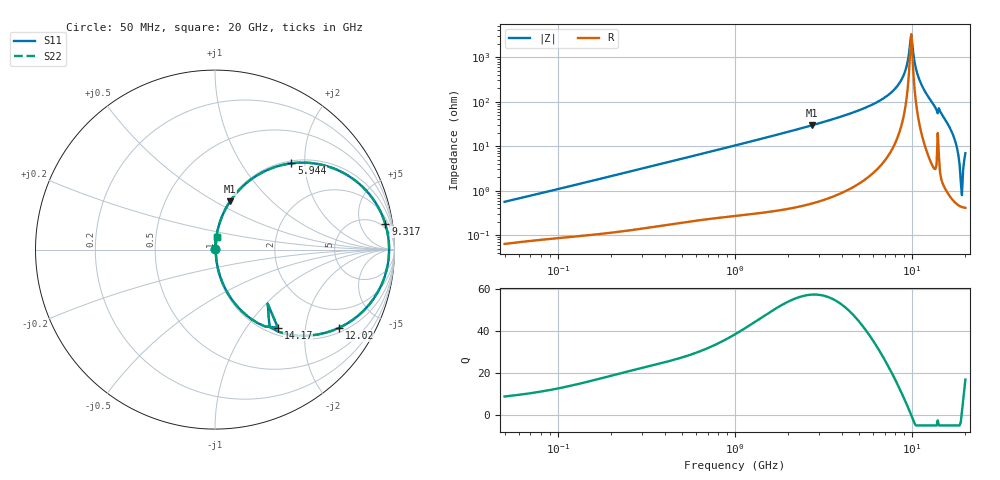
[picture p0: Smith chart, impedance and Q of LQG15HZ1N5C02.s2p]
!Murata Part Number: LQG15HZ1N5C02
!These Parameters are Measured in Series Mode Connection
!  o--[Z]--o
!Port1  Port2
!  o-------o
!Freq. Start=50[MHz] Stop=20[GHz], 401[Steps]
# Hz S RI R 50
!Freq.(Hz) S11(Real) S11(Imag) S21(Real) S21(Imag) S12(Real) S12(Imag) S22(Real) S22(Imag)
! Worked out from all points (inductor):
!   401 points, 50 MHz to 20 GHz, reference 50 ohm
!   read as one part in series: L = 1.75 nH near 51.52 MHz
!   highest Q = 57.4 at 2.728 GHz (marker M1), where L = 1.73 nH
!   self-resonance near 9.745 GHz
!   S11 on the Smith chart (normalised r, x): 50 MHz: 1.00, +0.01; 5.944 GHz: 1.05, +1.71; 9.317 GHz: 3, +12; 12.02 GHz: 1.16, -3.05; 14.17 GHz: 1.13, -1.42; 20 GHz: 1.01, +0.14
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5e7  0.000666 0.00558  0.9993 -0.00558  0.9993 -0.00558  0.000666 0.00558
1.364002e8  0.00118 0.0146  0.9988 -0.0146  0.9988 -0.0146  0.00118 0.0146
3.721004e8  0.00311 0.0388  0.9969 -0.0388  0.9969 -0.0388  0.00311 0.0388
1e9  0.0132 0.1021  0.9868 -0.1021  0.9868 -0.1021  0.0132 0.1021
2.728004e9  0.0844 0.2694  0.9156 -0.2694  0.9156 -0.2694  0.0844 0.2694
4.275624e9  0.2112 0.3984  0.7888 -0.3984  0.7888 -0.3984  0.2112 0.3984
5.944466e9  0.4259 0.4808  0.5741 -0.4808  0.5741 -0.4808  0.4259 0.4808
7.442007e9  0.68 0.4445  0.32 -0.4445  0.32 -0.4445  0.68 0.4445
8.516016e9  0.8592 0.3098  0.1408 -0.3098  0.1408 -0.3098  0.8592 0.3098
9.316812e9  0.9492 0.1427  0.0508 -0.1427  0.0508 -0.1427  0.9492 0.1427
9.600142e9  0.9649 0.0732  0.0351 -0.0732  0.0351 -0.0732  0.9649 0.0732
9.892087e9  0.9702 -0.00158  0.0298 0.00158  0.0298 0.00158  0.9702 -0.00158
1.082228e10  0.9084 -0.2346  0.0916 0.2346  0.0916 0.2346  0.9084 -0.2346
1.201863e10  0.6902 -0.4363  0.3098 0.4363  0.3098 0.4363  0.6902 -0.4363
1.417136e10  0.3503 -0.4348  0.6497 0.4348  0.6497 0.4348  0.3503 -0.4348
1.573793e10  0.1096 -0.2989  0.8904 0.2989  0.8904 0.2989  0.1096 -0.2989
1.721783e10  0.0301 -0.1538  0.9699 0.1538  0.9699 0.1538  0.0301 -0.1538
1.800918e10  0.0118 -0.0828  0.9882 0.0828  0.9882 0.0828  0.0118 -0.0828
1.855685e10  0.00588 -0.0372  0.9941 0.0372  0.9941 0.0372  0.00588 -0.0372
1.88369e10  0.00458 -0.0151  0.9954 0.0151  0.9954 0.0151  0.00458 -0.0151
1.940974e10  0.00496 0.0278  0.995 -0.0278  0.995 -0.0278  0.00496 0.0278
2e10  0.00887 0.0687  0.9911 -0.0687  0.9911 -0.0687  0.00887 0.0687
